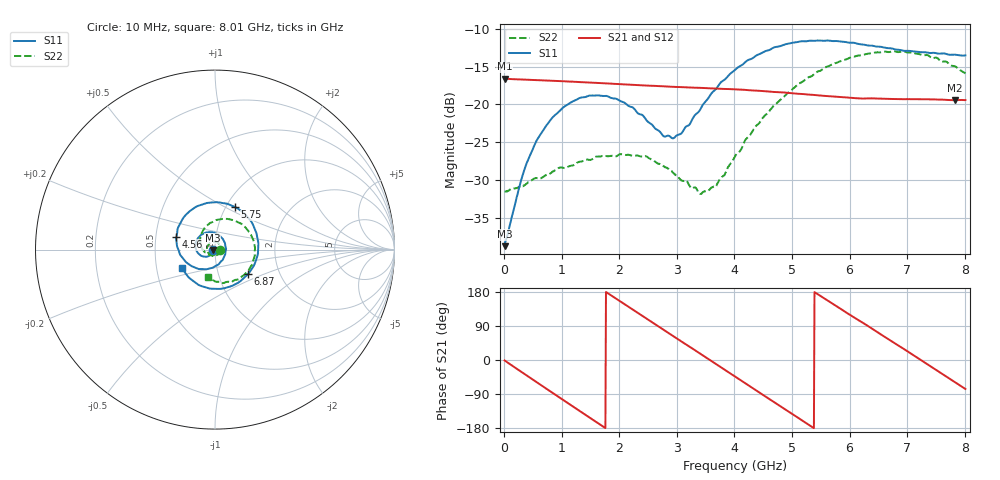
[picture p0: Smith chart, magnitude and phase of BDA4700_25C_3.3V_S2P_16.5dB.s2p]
!Agilent Technologies,E5071B,MY42404982,A.09.10
!Date: Mon Oct 20 18:09:58 2025
!Data & Calibration Information:
!Freq	S11:SOLT2(ON)	S21:SOLT2(ON)	S12:SOLT2(ON)	S22:SOLT2(ON)
# Hz S RI R 50
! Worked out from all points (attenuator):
!   801 points, 10 MHz to 8.01 GHz, reference 50 ohm
!   highest |S21| = -16.59 dB at 10 MHz (marker M1); lowest = -19.4 dB at 7.83 GHz (marker M2)
!   lowest |S11| = -38.7 dB at 10 MHz (marker M3), VSWR 1.02, Z = 48.9 - j0.157 ohm
!   |S11| at or under -10 dB: start of sweep to end of sweep
!   |S22| runs from -31.8 to -13.0 dB; largest |S21 - S12| = 0.0017
!   S11 on the Smith chart (normalised r, x): 10 MHz: 0.98, -0.00; 4.56 GHz: 0.64, +0.09; 5.75 GHz: 1.10, +0.56; 6.87 GHz: 1.38, -0.40; 8.01 GHz: 0.68, -0.15
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1e7  -0.0115 -0.0016  0.1481 -0.00319  0.1479 -0.00332  0.0266 -0.000825
3.3e8  -0.0223 -0.0267  0.1205 -0.0824  0.1203 -0.0823  0.0232 -0.017
5.6e8  -0.0421 -0.0387  0.0769 -0.1226  0.0769 -0.1226  0.0151 -0.0289
8.7e8  -0.0765 -0.0344  0.0012 -0.1431  0.00131 -0.1431  -0.00698 -0.0358
1.35e9  -0.1095 0.0195  -0.1046 -0.0934  -0.1046 -0.0936  -0.0383 -0.0172
1.97e9  -0.0525 0.0944  -0.1275 0.0483  -0.1276 0.0484  -0.0335 0.0314
2.45e9  0.0278 0.0759  -0.0485 0.124  -0.0486 0.1241  0.00133 0.0456
2.68e9  0.0542 0.0399  0.00342 0.1321  0.00324 0.132  0.0176 0.0366
2.96e9  0.058 -0.0167  0.0636 0.1139  0.0635 0.1138  0.0291 0.019
3.42e9  -0.00304 -0.0946  0.124 0.0338  0.1242 0.0338  0.0191 -0.0171
3.68e9  -0.0646 -0.1087  0.125 -0.0233  0.1251 -0.0237  -0.000782 -0.0288
4.01e9  -0.1491 -0.0792  0.0912 -0.0867  0.0913 -0.0865  -0.036 -0.0273
4.56e9  -0.215 0.0702  -0.0181 -0.1206  -0.0179 -0.1207  -0.0809 0.0306
4.93e9  -0.1682 0.187  -0.0848 -0.0837  -0.0845 -0.0843  -0.0735 0.0939
5.35e9  -0.0367 0.2606  -0.1156 -0.00633  -0.1155 -0.00701  -0.0135 0.1538
5.75e9  0.1124 0.2368  -0.0912 0.066  -0.091 0.0661  0.0789 0.1698
6.23e9  0.2285 0.0976  -0.0154 0.1082  -0.0139 0.1085  0.1844 0.1053
6.68e9  0.2228 -0.0749  0.0637 0.0883  0.0639 0.0882  0.2217 -0.0102
6.87e9  0.1828 -0.1379  0.0877 0.0635  0.088 0.0628  0.2125 -0.0642
7.33e9  0.028 -0.2188  0.1067 -0.0172  0.1068 -0.0173  0.1353 -0.1631
7.83e9  -0.1454 -0.1559  0.0562 -0.0906  0.056 -0.0909  0.00333 -0.1786
8.01e9  -0.184 -0.1028  0.0251 -0.1039  0.0255 -0.1037  -0.0384 -0.1552
